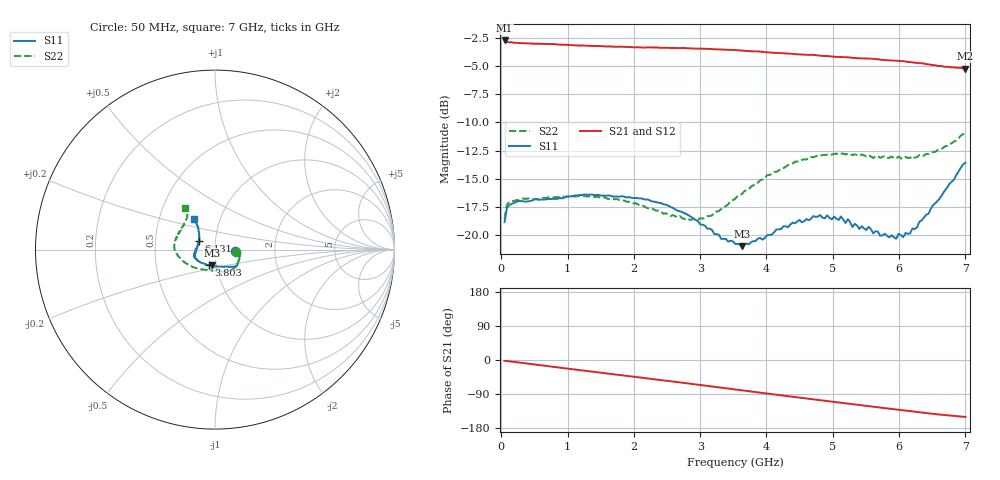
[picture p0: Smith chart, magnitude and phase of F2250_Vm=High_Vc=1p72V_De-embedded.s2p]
! Integrated Device Technology
! Corporate Headquarters
! 6024 Silver Creek Valley Road
! San Jose, CA 95138  USA
! Phone:  1-408-284-8200
! Toll Free:  1-800-223-1366
! Webpage:  http://www.idt.com/
! Timing and RF Division
! 515 Groton Road, Suite 102
! Westford, MA 01886-6024
! Device:  F2250
! Description: Voltage Variable RF Attenuator
! Frequency:  50.0 -  6000.00 MHz
! Package:  3x3 mm Thin QFN Plastic Package: 16 pin
! Ports:  2 RF, 3 DC
!  Pin  1  = GND
!  Pin  2  = NC
!  Pin  3  = RF1  = Port 1
!  Pin  4  = NC
!  Pin  5  = GND
!  Pin  6  = GND
!  Pin  7  = GND
!  Pin  8  = GND
!  Pin  9  = NC
!  Pin 10  = RF2  = Port 2
!  Pin 11  = NC
!  Pin 12  = GND
!  Pin 13  = GND
!  Pin 14  = VCNTRL
!  Pin 15  = VDD
!  Pin 16  = VMODE
! Vcntrl:  1.720 Volts
! Vmode:  +3.300 Volts
! Vdd:  +3.30  Volts
! Current:  1.326 mA
! Data:  The device was measured on a the F2250 evaluation board which has
!  individual transmission lines to the RF pins.  Data was collected
!  using a calibrated network analyzer.  The evaluation board was
!  de-embedded using a TRL calibration technique.
!  The reference plane is the edge of the package pin.
! Misc:  SN 10
!  Action Tracker AT0258
! Date Measured:  2014-11-26
! Date:  2015-10-15  MJV
! Note:
!  Integrated Device Technology supplies this data as a sample of measured
!  data at the package pin for this product.  Your particular data for this
!  product may vary.
!  Data was taken at 25 degrees C.
!  Integrated Device Technology reserves the right to change this data at anytime.
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# GHz S dB R 50
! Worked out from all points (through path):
!   201 points, 50 MHz to 7 GHz, reference 50 ohm
!   highest |S21| = -2.74 dB at 50 MHz (marker M1); lowest = -5.2 dB at 7 GHz (marker M2)
!   group delay of S21, straight-line fit = 60.4 ps
!   lowest |S11| = -21.0 dB at 3.629 GHz (marker M3), VSWR 1.20, Z = 47.8 - j8.51 ohm
!   |S11| at or under -10 dB: start of sweep to end of sweep
!   |S22| runs from -18.6 to -10.9 dB; largest |S21 - S12| = 0.0029
!   S11 on the Smith chart (normalised r, x): 50 MHz: 1.26, -0.03; 3.803 GHz: 0.92, -0.16; 6.131 GHz: 0.83, +0.08; 7 GHz: 0.75, +0.27
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0.05  -18.84 -5.0  -2.74 -2.1  -2.75 -2.1  -18.53 -6.1
0.08475  -17.59 -4.3  -2.87 -2.6  -2.88 -2.6  -17.30 -5.3
0.2585  -16.98 -9.1  -2.97 -6.4  -2.96 -6.4  -16.89 -12.1
1.2315  -16.42 -33.8  -3.18 -27.7  -3.19 -27.7  -16.54 -46.7
2.37825  -17.13 -43.3  -3.38 -52.1  -3.40 -52.2  -17.82 -72.4
2.969  -18.78 -55.5  -3.47 -65.2  -3.47 -65.2  -18.62 -99.7
3.525  -20.76 -90.8  -3.59 -77.7  -3.60 -77.7  -16.78 -134.1
3.62925  -20.97 -99.3  -3.64 -80.1  -3.63 -80.1  -16.35 -139.4
3.803  -20.53 -112.6  -3.71 -83.9  -3.71 -83.9  -15.57 -147.4
4.4285  -18.95 -146.2  -3.95 -97.7  -3.96 -97.7  -13.49 -171.1
4.7065  -18.30 -156.7  -4.02 -103.8  -4.03 -103.8  -13.10 -178.1
5.1235  -18.34 -167.2  -4.21 -112.8  -4.21 -112.9  -12.78 171.8
5.193  -18.92 -169.4  -4.23 -114.3  -4.22 -114.4  -12.85 170.3
5.22775  -18.58 -170.6  -4.23 -115.1  -4.23 -115.1  -12.77 169.5
5.29725  -19.28 -171.6  -4.28 -116.5  -4.26 -116.6  -12.91 168.2
5.5405  -19.26 178.8  -4.36 -121.8  -4.36 -121.9  -12.91 161.5
5.61  -19.84 179.0  -4.37 -123.3  -4.37 -123.3  -13.16 160.4
5.85325  -20.20 166.9  -4.50 -128.4  -4.50 -128.5  -13.15 153.2
6.13125  -19.87 150.8  -4.64 -134.3  -4.64 -134.5  -13.16 145.5
6.27025  -19.31 142.9  -4.73 -137.4  -4.71 -137.4  -13.08 140.7
6.54825  -17.16 132.1  -4.93 -142.8  -4.95 -142.9  -12.60 132.1
7  -13.58 124.8  -5.23 -150.3  -5.23 -150.4  -10.91 125.9
